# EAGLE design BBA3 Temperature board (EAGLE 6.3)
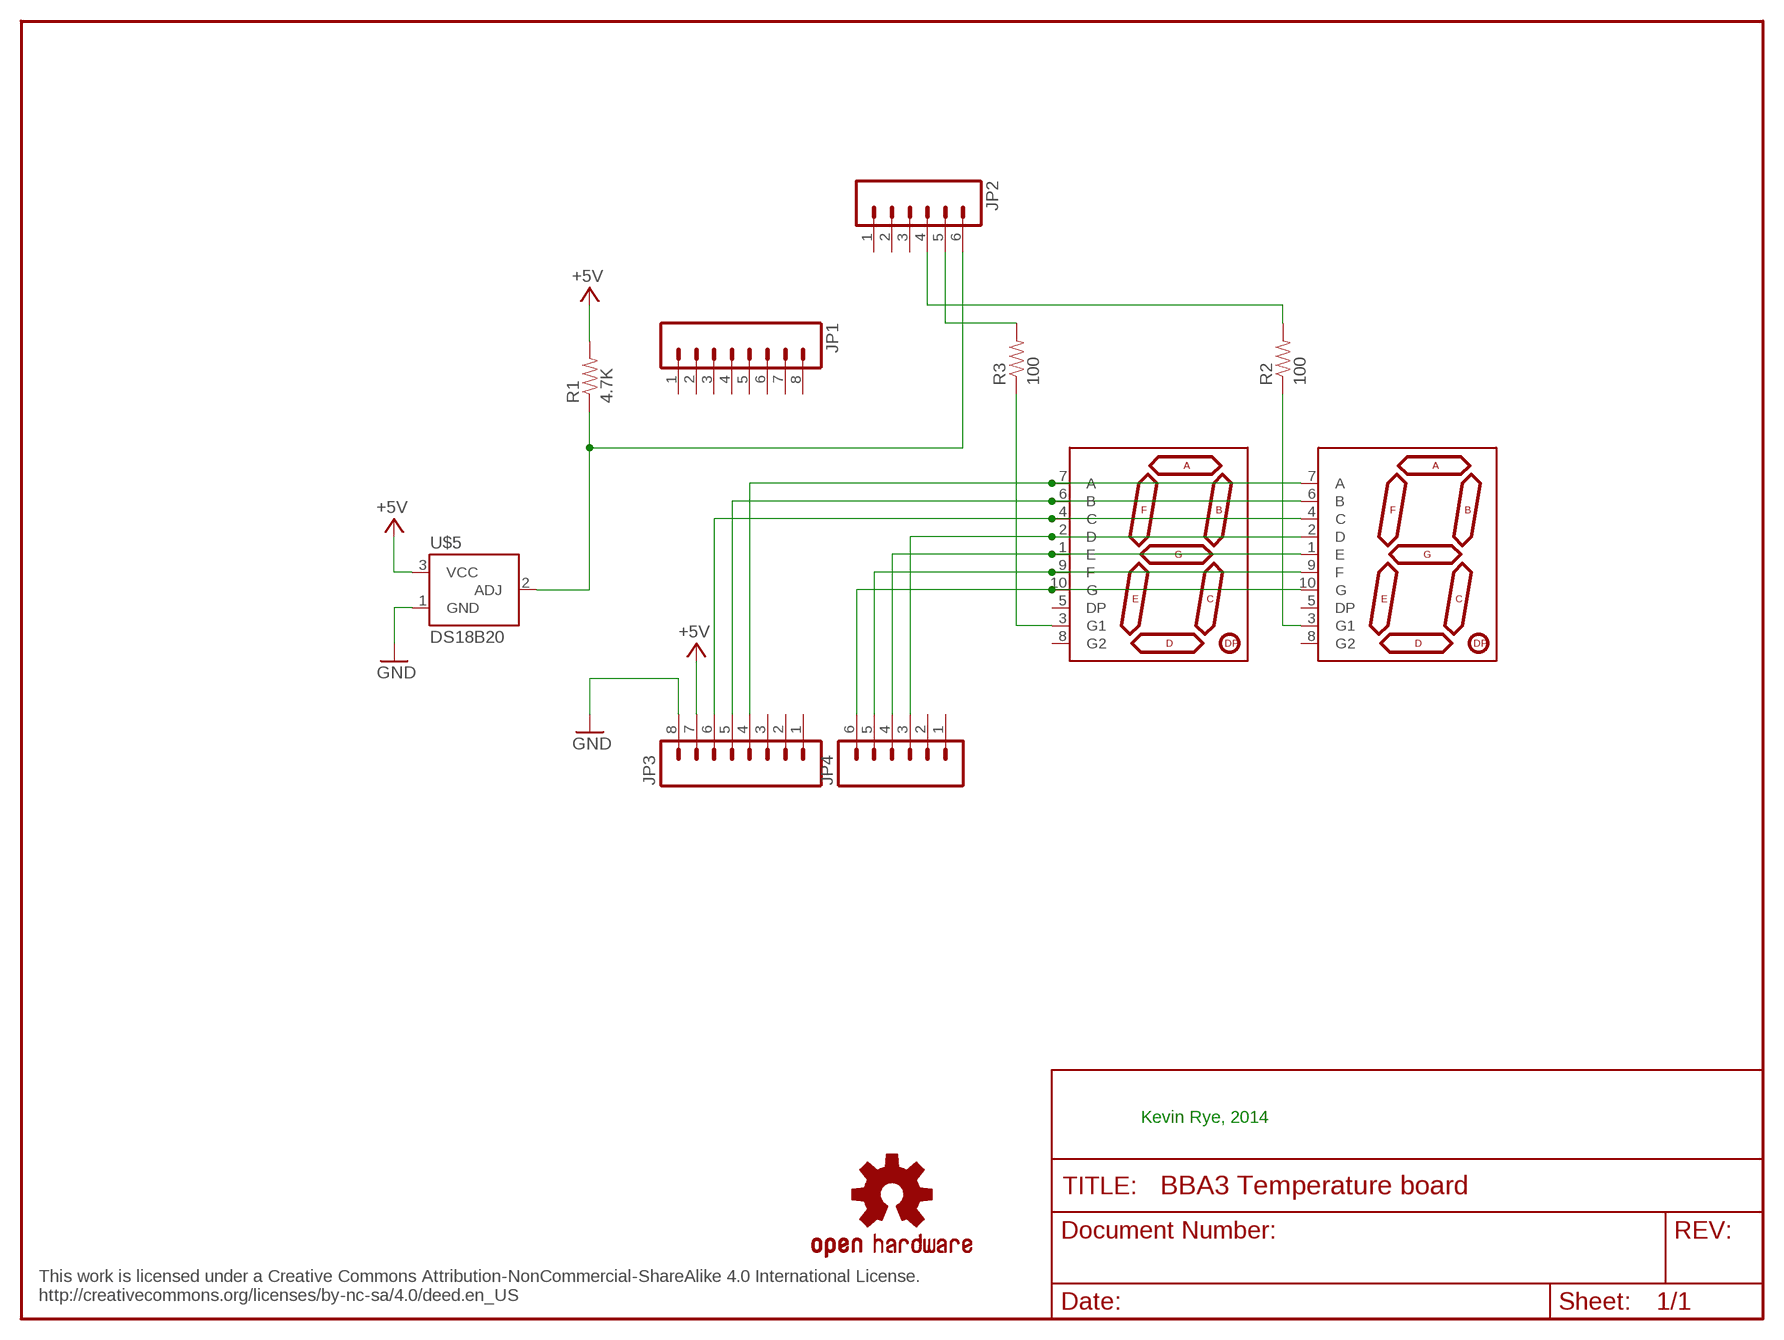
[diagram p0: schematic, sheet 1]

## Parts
DIGIT1  7-SEGMENT-DISPLAYPTH  [7-SEGMENT-DISPLAY]
JP1  M081X08  [1X08]
JP2  M06SIP  [1X06]
JP3  M081X08  [1X08]
JP4  M06SIP  [1X06]
R1  4.7K  RESISTOR0805-RES  [0805]
R2  100  RESISTOR0805-RES  [0805]
R3  100  RESISTOR0805-RES  [0805]
U$1  OSHW-LOGOS  [OSHW-LOGO-S]
U$4  7-SEGMENT-DISPLAYPTH  [7-SEGMENT-DISPLAY]
U$5  DS18B20  TEMPERATURE-SENSOR  [TO-92]

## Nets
+5V [power]: JP3.7 R1.2 U$5.3(VCC)
GND [power]: JP3.8 U$5.1(GND)
N$1: DIGIT1.7(A) JP3.4 U$4.7(A)
N$2: DIGIT1.6(B) JP3.5 U$4.6(B)
N$3: DIGIT1.4(C) JP3.6 U$4.4(C)
N$4: DIGIT1.2(D) JP4.3 U$4.2(D)
N$5: DIGIT1.1(E) JP4.4 U$4.1(E)
N$6: DIGIT1.9(F) JP4.5 U$4.9(F)
N$7: DIGIT1.10(G) JP4.6 U$4.10(G)
N$8: DIGIT1.3(G1) R3.1
N$9: R2.1 U$4.3(G1)
N$10: JP2.6 R1.1 U$5.2(ADJ)
N$11: JP2.5 R3.2
N$12: JP2.4 R2.2
Unconnected: DIGIT1.5(DP) DIGIT1.8(G2) JP1.1 JP1.2 JP1.3 JP1.4 JP1.5 JP1.6 JP1.7 JP1.8 JP2.1 JP2.2 JP2.3 JP3.1 JP3.2 JP3.3 JP4.1 JP4.2 U$4.5(DP) U$4.8(G2)

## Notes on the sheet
- Kevin Rye, 2014
- This work is licensed under a Creative Commons Attribution-NonCommercial-ShareAlike 4.0 International License.
  http://creativecommons.org/licenses/by-nc-sa/4.0/deed.en_US

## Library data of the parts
DIGIT1 U$4 = SparkFun-Displays:7-SEGMENT-DISPLAY
JP1 JP3 = SparkFun:M08: Header 8 Standard 8-pin 0.1" header. Use with straight break away headers (SKU : PRT-00116), right angle break away headers (PRT-00553), swiss pins (PRT-00743), machine pins (PRT-00117), and female headers (PRT-00115).
JP2 JP4 = SparkFun:M06: Header 6 Standard 6-pin 0.1" header. Use with straight break away headers (SKU : PRT-00116), right angle break away headers (PRT-00553), swiss pins (PRT-00743), machine pins (PRT-00117), and female headers (PRT-00115). Molex polarized connector foot print use with SKU : PRT-08094 with associated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
R1-R3 = SparkFun-Resistors:RESISTOR: Resistor
U$1 = SparkFun:OSHW-LOGO: Open Source Hardware Logo This logo indicates the piece of hardware it is found on incorporates a OSHW license and/or adheres to the definition of open source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
U$5 = SparkFun-Sensors:TEMPERATURE-SENSOR: TO-92 temp sensor

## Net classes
0 default: width 0.4 mm, clearance 0.3 mm
1 power: width 0.6 mm, clearance 0.3 mm

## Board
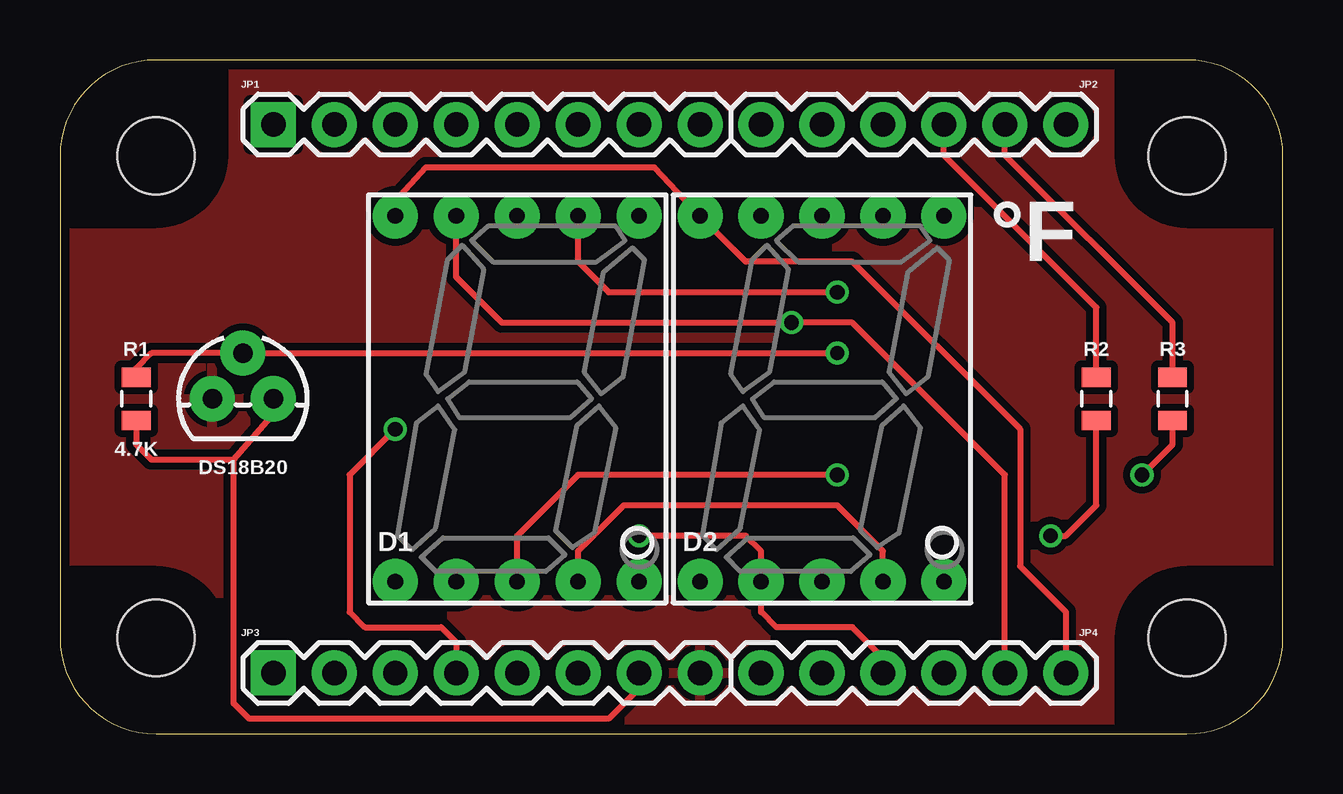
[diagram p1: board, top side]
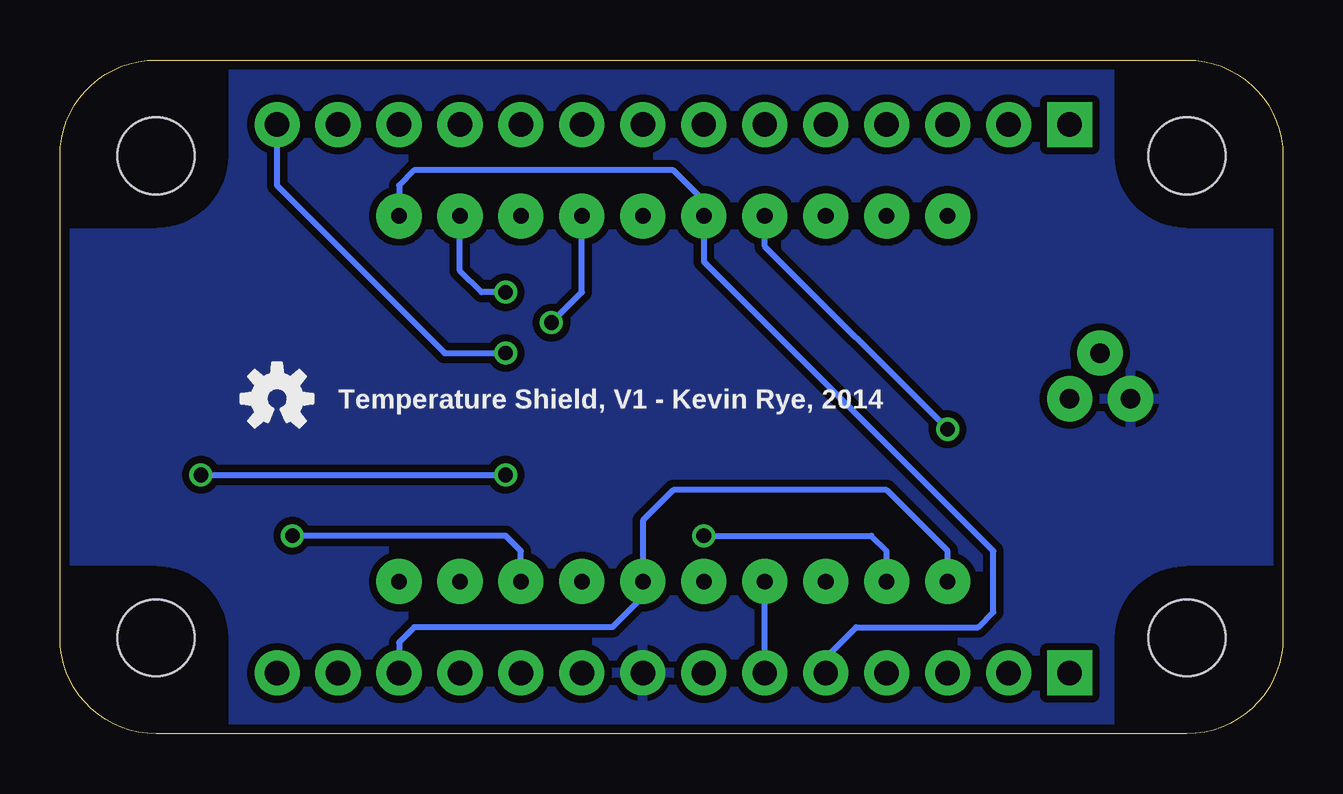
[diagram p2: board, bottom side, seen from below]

Size 50.95 x 28.09 mm. Coordinates in mm from the lower left corner, seen from the top.
Copper layers (1*16): Top 0.0356mm / dielectric 1.5011mm / Bottom 0.0356mm
Design rules "LaenPCBOrder": minimum track width 6mil, minimum drill 13mil, track to track 6mil, track to pad 6mil, pad to pad 6mil, via to via 6mil, smd to smd 6mil, copper to edge 15mil, drill to drill 6mil, minimum pad ring 7mil, minimum via ring 7mil, stop-mask expansion 3mil, vias tented up to drill 0mil, thermal gap 10mil

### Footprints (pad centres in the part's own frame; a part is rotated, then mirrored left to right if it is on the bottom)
7-SEGMENT-DISPLAY = drill 0.65 pad 1.88: 1 -5.08,-7.62; 2 -2.54,-7.62; 3 0,-7.62; 4 2.54,-7.62; 5 5.08,-7.62; 6 5.08,7.62; 7 2.54,7.62; 8 0,7.62; 9 -2.54,7.62; 10 -5.08,7.62
1X08 = drill 1.016 pad 1.88 square: 1 0,0 | drill 1.016 pad 1.88: 2 2.54,0; 3 5.08,0; 4 7.62,0; 5 10.16,0; 6 12.7,0; 7 15.24,0; 8 17.78,0
1X06 = drill 1.016 pad 1.88: 1 0,0; 2 2.54,0; 3 5.08,0; 4 7.62,0; 5 10.16,0; 6 12.7,0
0805 = smd 0.8 x 1.2: 1 -0.9,0; 2 0.9,0
2.2X1 = hole 3.2: 4,4; 46.955,4; 46.955,24.095; 4,24.095
TO-92 = drill 0.813 pad 1.88: 1 -1.27,0; 2 0,1.905; 3 1.27,0

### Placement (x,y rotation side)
DIGIT1  19.05,13.97 0 top
JP1  8.89,25.4 0 top
JP2  29.21,25.4 0 top
JP3  8.89,2.54 0 top
JP4  29.21,2.54 0 top
R1  3.18,13.97 270 top
R2  43.18,13.97 90 top
R3  46.36,13.97 90 top
U$1  41.91,13.97 0 bottom
U$2  [2.2X1]  0,0 0 top
U$4  31.75,13.97 0 top
U$5  7.62,13.97 0 top

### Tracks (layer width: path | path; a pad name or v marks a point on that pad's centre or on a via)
+5V
  Top 0.254: JP3.7 24.13,1.91 22.86,0.64 7.88,0.64 7.24,1.27 7.24,11.43 | 7.24,11.43 8.89,13.34 U$5.3 | R1.2 3.18,12.06 3.81,11.43 7.24,11.43
GND
  pour Top: -2.54,32.38 53.97,33.66 53.97,-0.64 -2.54,-0.64
  pour Bottom: -1.91,32.38 53.34,33.02 52.7,-0.64 -1.91,-1.27
N$1  (via drill 0.61)
  Top 0.254: v32.38,18.41 22.86,18.41 21.59,19.68 DIGIT1.7 | v13.97,12.7 12.06,10.79 12.06,5.08 12.7,4.45 15.88,4.45 16.51,3.81 JP3.4
  Bottom 0.254: v13.97,12.7 21.59,20.32 DIGIT1.7 | v32.38,18.41 33.39,18.41 34.29,19.31 U$4.7
N$2
  Bottom 0.254: U$4.6 36.83,22.86 36.2,23.5 25.4,23.5 24.13,22.23 DIGIT1.6 24.13,19.68 12.06,7.62 12.06,5.08 12.7,4.45 17.78,4.45 19.05,3.17 JP3.5
N$3
  Top 0.254: U$4.4 34.29,7.62 32.38,9.53 23.49,9.53 21.59,7.62 DIGIT1.4
  Bottom 0.254: JP3.6 DIGIT1.4
N$4  (via drill 0.61)
  Top 0.254: JP4.3 34.29,3.17 33.02,4.45 29.84,4.45 29.21,5.08 U$4.2 29.21,7.62 28.58,8.26 v24.13,8.26
  Bottom 0.254: DIGIT1.2 16.51,7.62 17.15,8.26 v24.13,8.26
N$5
  Bottom 0.254: JP4.4 36.83,3.81 36.2,4.45 27.94,4.45 26.67,5.71 U$4.1 26.67,8.89 25.4,10.16 16.51,10.16 13.97,7.62 DIGIT1.1
N$6  (via drill 0.61)
  Top 0.254: JP4.5 39.37,10.79 33.02,17.14 v30.48,17.14 18.41,17.14 16.51,19.05 DIGIT1.9
  Bottom 0.254: v30.48,17.14 29.21,18.41 U$4.9
N$7
  Top 0.254: DIGIT1.10 13.97,22.23 15.24,23.62 24.77,23.62 U$4.10 28.58,19.68 33.02,19.68 40.01,12.7 40.01,6.99 41.91,5.08 JP4.6
N$8  (via drill 0.61)
  Top 0.254: v32.38,10.79 21.59,10.79 19.05,8.26 DIGIT1.3 | v45.08,10.79 46.36,12.06 R3.1
  Bottom 0.254: v45.08,10.79 v32.38,10.79
N$9  (via drill 0.6)
  Top 0.254: v41.28,8.26 41.91,8.26 43.18,9.53 R2.1
  Bottom 0.254: U$4.3 31.75,7.62 32.38,8.26 v41.28,8.26
N$10  (via drill 0.6)
  Top 0.254: R1.1 3.18,15.24 3.81,15.88 U$5.2 v32.38,15.88
  Bottom 0.254: v32.38,15.88 34.92,15.88 41.91,22.86 JP2.6
N$11
  Top 0.254: R3.2 46.36,17.14 39.37,24.13 JP2.5
N$12
  Top 0.254: R2.2 43.18,17.78 36.83,24.13 JP2.4

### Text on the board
Unrouted: This work is licensed under a Creative Commons Attribution-NonCommercial-ShareAlike 4.0 International License. / http://creativecommons.org/licenses/by-nc-sa/4.0/deed.en_US
tNames: °F | D1 | D2
bNames: Temperature Shield, V1 - Kevin Rye, 2014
